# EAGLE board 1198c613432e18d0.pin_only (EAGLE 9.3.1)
REV: F

Size 85.72 x 54.1 mm. Coordinates in mm from the lower left corner, seen from the top.
Outline: 0,51.05 0,3.17 arc90 3.05,0 82.68,0 arc90 85.72,3.17 85.72,51.05 arc90 82.68,54.1 60.77,54.1 59.37,52.71 56.07,52.71 54.67,54.1 3.05,54.1 arc90 0,51.05
Copper layers (1*16): Top 0.035mm / dielectric 1.5mm / Bottom 0.035mm
Design rules "adafruit *": minimum track width 8mil, minimum drill 19mil, track to track 8mil, track to pad 8mil, pad to pad 8mil, via to via 8mil, smd to smd 8mil, copper to edge 10mil, drill to drill 8mil, minimum pad ring 10mil, minimum via ring 8mil, stop-mask expansion 2mil, vias tented up to drill 20mil, thermal gap 10mil
Net classes: 1 power: width 0.305 mm; 2 gnd: width 0.254 mm

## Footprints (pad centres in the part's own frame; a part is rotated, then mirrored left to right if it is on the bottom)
6MM_SMT = smd 2 x 1.2: A -3.3,-2.2; A' 3.3,-2.2; B -3.3,2.2; B' 3.3,2.2
0603-NO = smd 1.075 x 1: 1 -0.85,0; 2 0.85,0
0805-NO = smd 1.24 x 1.5: 1 -0.95,0; 2 0.95,0
_0805MP = smd 1.2 x 1.3: 1 -1.016,0; 2 1.016,0
CHIPLED_0805_NOOUTLINE = smd 1.2 x 1.2: A 0,-1.05; C 0,1.05
SOD-323 = smd 1.35 x 0.8: A 1.27,0; C -1.27,0
SOD-123 = smd 1.4 x 1.4: A 1.85,0; C -1.85,0
JSTPH4 = smd 1 x 4.6: 1 -3,-3.7; 2 -1,-3.7; 3 1,-3.7; 4 3,-3.7 | smd 1.7 x 3.4: NC1 -5.7,1.5; NC2 5.7,1.5
TSSOP16 = smd 0.305 x 0.991: 1 -2.275,-2.918; 2 -1.625,-2.918; 3 -0.975,-2.918; 4 -0.325,-2.918; 5 0.325,-2.918; 6 0.975,-2.918; 7 1.625,-2.918; 8 2.275,-2.918; 9 2.275,2.918; 10 1.625,2.918; 11 0.975,2.918; 12 0.325,2.918; 13 -0.325,2.918; 14 -0.975,2.918; 15 -1.625,2.918; 16 -2.275,2.918
SOT23-6 = smd 0.55 x 1.2: 1 -0.95,-1.3; 2 0,-1.3; 3 0.95,-1.3; 4 0.95,1.3; 5 0,1.3; 6 -0.95,1.3
LGA16_3X3MM = smd 0.5 x 0.25: 1 -1.35,1; 2 -1.35,0.5; 3 -1.35,0; 4 -1.35,-0.5; 5 -1.35,-1; 9 1.35,-1; 10 1.35,-0.5; 11 1.35,0; 12 1.35,0.5; 13 1.35,1 | smd 0.25 x 0.5: 6 -0.5,-1.35; 7 0,-1.35; 8 0.5,-1.35; 14 0.5,1.35; 15 0,1.35; 16 -0.5,1.35
JD-T1800 = smd 0.5 x 2: 1 5.2,-13.1; 2 4.4,-13.1; 3 3.6,-13.1; 4 2.8,-13.1; 5 2,-13.1; 6 1.2,-13.1; 7 0.4,-13.1; 8 -0.4,-13.1; 9 -1.2,-13.1; 10 -2,-13.1; 11 -2.8,-13.1; 12 -3.6,-13.1; 13 -4.4,-13.1; 14 -5.2,-13.1 | hole 0.6: -12.8,-16.9; 7.65,-16.9
LED3535 = smd 1 x 0.85: 1 -1.75,0.875; 2 -1.75,-0.875; 3 1.75,-0.875; 4 1.75,0.875
FEATHERWING_SMT_NOHOLES = smd 1.524 x 2.54: 1 6.35,2.413; 1B 6.35,-2.413; 2 8.89,2.413; 2B 8.89,-2.413; 15 41.91,2.413; 15B 41.91,-2.413; 16 44.45,2.413; 16B 44.45,-2.413; 17 44.45,20.447; 17B 44.45,25.273; 18 41.91,20.447; 18B 41.91,25.273; 27 19.05,20.447; 27B 19.05,25.273; 28 16.51,20.447; 28B 16.51,25.273 | smd 1.524 x 3.048: 3 11.43,2.159; 3B 11.43,-2.159; 4 13.97,2.159; 4B 13.97,-2.159; 5 16.51,2.159; 5B 16.51,-2.159; 6 19.05,2.159; 6B 19.05,-2.159; 7 21.59,2.159; 7B 21.59,-2.159; 8 24.13,2.159; 8B 24.13,-2.159; 9 26.67,2.159; 9B 26.67,-2.159; 10 29.21,2.159; 10B 29.21,-2.159; 11 31.75,2.159; 11B 31.75,-2.159; 12 34.29,2.159; 12B 34.29,-2.159; 13 36.83,2.159; 13B 36.83,-2.159; 14 39.37,2.159; 14B 39.37,-2.159; 19 39.37,20.701; 19B 39.37,25.019; 20 36.83,20.701; 20B 36.83,25.019; 21 34.29,20.701; 21B 34.29,25.019; 22 31.75,20.701; 22B 31.75,25.019; 23 29.21,20.701; 23B 29.21,25.019; 24 26.67,20.701; 24B 26.67,25.019; 25 24.13,20.701; 25B 24.13,25.019; 26 21.59,20.701; 26B 21.59,25.019
JSTPH3 = smd 1 x 4.6: 1 -2,-2.7; 2 0,-2.7; 3 2,-2.7 | smd 1.6 x 3.4: NC1 -4.4,2.5; NC2 4.4,2.5
SOT23-R = smd 0.635 x 1.016: 1 -0.95,-1; 2 0.95,-1; 3 0,1
SOT23-WIDE = smd 1 x 1.2: 1 -0.95,-1; 2 0.95,-1; 3 0,1
SOT363 = smd 0.5 x 0.5: 1 -0.75,-0.9; 3 0.75,-0.9; 4 0.75,0.9; 6 -0.75,0.9 | smd 0.4 x 0.5: 2 0,-0.9; 5 0,0.9
RESPACK_4X0603 = smd 0.45 x 0.9: 1 -1.3,-0.85; 2 -0.4,-0.85; 3 0.4,-0.85; 4 1.3,-0.85; 5 1.3,0.85; 6 0.4,0.85; 7 -0.4,0.85; 8 -1.3,0.85
SOLDERJUMPER_2WAY_OPEN_NOPASTE = smd 1.168 x 1.6: 1 -1.397,0; 2 0,0; 3 1.397,0
SOLDERJUMPER_CLOSEDWIRE = smd 1.168 x 1.6: 1 -0.762,0; 2 0.762,0 | smd 0.635 x 0.203: WIRE 0,0
BUZZER_SMT_7.5MM = smd 2 x 2: + 2.8,-2.8; - 2.8,2.8; MT2 -2.8,2.8 | smd 2 x 1 rotated 135: MT -3,-3
EVQ-Q2_SMALLER = smd 2 x 1.2: A -3.1,-2; A' 3.1,-2; B -3.1,2; B' 3.1,2
SPDT_SMT_SSSS811101 = smd 0.7 x 1.5: A -2.25,1.75; B 0.75,1.75; C 2.25,1.75 | smd 1 x 0.8: SUP1 -3.65,1.1; SUP2 -3.65,-1.1; SUP3 3.65,1.1; SUP4 3.65,-1.1 | hole 0.9: -1.5,0; 1.5,0
TESTPOINT_ROUND_2MM = smd 2 x 2: P$1 0,0
SOIC8_208MIL = smd 0.6 x 2.2: 1 -1.905,-3.315; 2 -0.635,-3.315; 3 0.635,-3.315; 4 1.905,-3.315; 5 1.905,3.315; 6 0.635,3.315; 7 -0.635,3.315; 8 -1.905,3.315
SOT23-5 = smd 0.55 x 1.2: 1 -0.95,-1.3; 2 0,-1.3; 3 0.95,-1.3; 4 0.95,1.3; 5 -0.95,1.3
ALS-PT26-21C = smd 1.5 x 1.6: 1_E -1.8,0; 2_C 1.8,0 | hole 2.4: 0,0
MOUNTINGHOLE_3.0_PLATEDTHIN = drill 3 pad 3.6: P$1 0,0
53398-0271 = smd 0.8 x 1.6: 1 0.625,-1.27; 2 -0.625,-1.27 | smd 2.1 x 3: M1 3.185,1.48; M2 -3.185,1.48
PQFN64-1 = smd 0.7 x 0.22: 1 -4.45,3.75; 2 -4.45,3.25; 3 -4.45,2.75; 4 -4.45,2.25; 5 -4.45,1.75; 6 -4.45,1.25; 7 -4.45,0.75; 8 -4.45,0.25; 9 -4.45,-0.25; 10 -4.45,-0.75; 11 -4.45,-1.25; 12 -4.45,-1.75; 13 -4.45,-2.25; 14 -4.45,-2.75; 15 -4.45,-3.25; 16 -4.45,-3.75; 33 4.45,-3.75; 34 4.45,-3.25; 35 4.45,-2.75; 36 4.45,-2.25; 37 4.45,-1.75; 38 4.45,-1.25; 39 4.45,-0.75; 40 4.45,-0.25; 41 4.45,0.25; 42 4.45,0.75; 43 4.45,1.25; 44 4.45,1.75; 45 4.45,2.25; 46 4.45,2.75; 47 4.45,3.25; 48 4.45,3.75 | smd 0.22 x 0.7: 17 -3.75,-4.45; 18 -3.25,-4.45; 19 -2.75,-4.45; 20 -2.25,-4.45; 21 -1.75,-4.45; 22 -1.25,-4.45; 23 -0.75,-4.45; 24 -0.25,-4.45; 25 0.25,-4.45; 26 0.75,-4.45; 27 1.25,-4.45; 28 1.75,-4.45; 29 2.25,-4.45; 30 2.75,-4.45; 31 3.25,-4.45; 32 3.75,-4.45; 49 3.75,4.45; 50 3.25,4.45; 51 2.75,4.45; 52 2.25,4.45; 53 1.75,4.45; 54 1.25,4.45; 55 0.75,4.45; 56 0.25,4.45; 57 -0.25,4.45; 58 -0.75,4.45; 59 -1.25,4.45; 60 -1.75,4.45; 61 -2.25,4.45; 62 -2.75,4.45; 63 -3.25,4.45; 64 -3.75,4.45 | smd 4.7 x 4.7: EXP 0,0
FIDUCIAL_1MM = smd 1 x 1: 1 0,0
JSTPH2 = smd 1 x 4.6: 1 -1,-3.7; 2 1,-3.7 | smd 1.6 x 3.4: NC1 -3.4,1.5; NC2 3.4,1.5
2X05_1.27MM_BOX_POSTS = smd 0.76 x 2.6: 1 -2.54,-2.15; 2 -2.54,2.15; 3 -1.27,-2.15; 4 -1.27,2.15; 5 0,-2.15; 6 0,2.15; 7 1.27,-2.15; 8 1.27,2.15; 9 2.54,-2.15; 10 2.54,2.15 | hole 1: -1.905,0; 1.905,0
4UCONN_20329_V2 = smd 1 x 2: BASE@1 -0.75,-2; BASE@2 0.75,-2 | smd 0.4 x 1.35: D+ 0,0.775; D- -0.65,0.775; GND 1.3,0.775; ID 0.65,0.775; VBUS -1.3,0.775 | drill 0.8 pad 1.143 offset: SPRT@1 -3.3,0.9; SPRT@2 3.3,0.9 | drill 0.9 pad 2.413 square: SPRT@3 -3.6,-1.9; SPRT@4 3.6,-1.9 | hole 0.7: -1.95,0; 1.95,0

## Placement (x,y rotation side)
A  [6MM_SMT]  5.14,34.93 270 bottom
B  [6MM_SMT]  12.83,30.04 270 bottom
C1  1uF  [0603-NO]  77.47,52.77 0 top
C2  1uF  [0603-NO]  48.64,9.08 0 top
C3  10µF  [0805-NO]  42.29,37.21 180 top
C4  1uF  [0603-NO]  26.35,16.26 90 top
C5  10uF  [0805-NO]  36.51,45.21 270 top
C6  10µF  [0805-NO]  41.72,44.39 180 top
C7  1uF  [0603-NO]  44.66,38.34 90 top
C8  10µF  [0805-NO]  45.23,35.12 270 top
C9  0.1uF  [0603-NO]  17.97,45.34 180 top
C10  10uF  [0805-NO]  68.01,2.16 0 top
C11  10uF  [0805-NO]  26.23,30.72 270 top
C12  1uF  [0603-NO]  37.08,19.49 180 top
C13  1uF  [0603-NO]  26.42,41.66 270 top
C14  10uF  [0805-NO]  48.7,17.34 270 top
C15  10uF  [0805-NO]  16.51,52.64 0 top
C16  10µF  [_0805MP]  25.55,36.78 180 top
C17  0.1uF  [0603-NO]  23.81,12.89 0 top
C18  10uF  [0805-NO]  42.1,35.37 180 top
C19  1uF  [0603-NO]  42.16,33.85 180 top
CHG  ORANGE  [CHIPLED_0805_NOOUTLINE]  36.58,52.07 180 top
D1  3.6V  [SOD-323]  24.51,10.54 0 top
D2  3.6V  [SOD-323]  68.26,5.78 270 top
D4  MBR0540  [SOD-123]  46.48,47.12 0 top
DOWN  [6MM_SMT]  74.93,27.18 45 bottom
FB1  Ferrite  [0805-NO]  26.48,44.96 270 top
I2C  JST PH 4  [JSTPH4]  42.86,3.49 180 top
IC1  74165TSSOP  [TSSOP16]  71.69,50.23 270 top
IC2  PAM8301  [SOT23-6]  16.19,49.72 0 top
IC4  LIS3DH  [LGA16_3X3MM]  47.75,11.75 180 top
L  RED  [CHIPLED_0805_NOOUTLINE]  48.98,51.97 0 top
LCD1  DISP_LCD_JDT1800  [JD-T1800]  40.13,28.83 90 bottom
LED1  WS2812B3535  [LED3535]  60.33,6.48 0 bottom
LED2  WS2812B3535  [LED3535]  51.59,6.48 0 bottom
LED3  WS2812B3535  [LED3535]  42.86,6.48 0 bottom
LED4  WS2812B3535  [LED3535]  34.13,6.48 0 bottom
LED5  WS2812B3535  [LED3535]  25.4,6.48 0 bottom
LEFT  [6MM_SMT]  80.2,32.51 315 bottom
MS1  FEATHERWING_SMTDUALNOHOLES  [FEATHERWING_SMT_NOHOLES]  31.43,54.1 270 top
NEOPIX  JST PH 3  [JSTPH3]  24.64,4.51 180 top
Q1  DMG3405  [SOT23-R]  45.85,41.66 180 top
Q2  DMG3405  [SOT23-R]  45.85,44.45 180 top
Q3  BSS138  [SOT23-WIDE]  24.08,34.24 90 top
Q4  BSS138  [SOT363]  53.53,3.56 0 top
R1  100K  [RESPACK_4X0603]  47.62,34.04 90 top
R2  1K  [0603-NO]  36.58,48.77 270 top
R3  10K  [0603-NO]  28,49.85 0 top
R4  10K  [RESPACK_4X0603]  53.59,6.54 0 top
R5  1K  [0603-NO]  21.15,9.72 90 top
R6  1K  [0603-NO]  66.93,6.6 90 top
R7  2.2K  [0603-NO]  50.04,49.02 180 top
R8  4.7K  [0603-NO]  41.59,42.86 0 top
R9  DNP  [0603-NO]  52.58,9.14 0 bottom
R10  100K  [RESPACK_4X0603]  77.47,50.04 270 top
R11  100K  [RESPACK_4X0603]  66.48,50.29 90 top
R12  47K  [0603-NO]  17.59,46.86 0 top
R14  10K  [0603-NO]  24.7,15.24 270 top
R15  10K  [0603-NO]  26.29,12.83 270 top
R16  10  [0603-NO]  23.62,30.99 90 top
R17  100K  [0603-NO]  26.45,34.12 90 top
R19  100K  [0603-NO]  37.08,17.97 180 top
RIGHT  [6MM_SMT]  69.66,32.51 135 bottom
SELECT  [6MM_SMT]  73.22,50.42 180 bottom
SENSE  JST PH 3  [JSTPH3]  61.02,4.51 180 top
SJ1  [SOLDERJUMPER_2WAY_OPEN_NOPASTE]  70.87,4.25 270 top
SJ2  [SOLDERJUMPER_CLOSEDWIRE]  13.84,44.58 180 top
SP1  SPEAKER_7.5MM  [BUZZER_SMT_7.5MM]  10.16,49.59 270 top
START  [6MM_SMT]  12.76,50.42 180 bottom
SW1  SPST_TACT-EVQQ2  [EVQ-Q2_SMALLER]  22.48,50.48 0 top
SW11  [SPDT_SMT_SSSS811101]  57.78,51.24 180 top
TP6  [TESTPOINT_ROUND_2MM]  9.91,10.73 0 top
TP7  [TESTPOINT_ROUND_2MM]  5.14,10.79 0 top
TP8  [TESTPOINT_ROUND_2MM]  13.65,10.86 0 top
U1  GD25Q16  [SOIC8_208MIL]  40.26,13.72 270 top
U2  AP2112-3.3  [SOT23-5]  47.37,38.23 90 top
U3  MCP73831T-2ACI/OT  [SOT23-5]  42.29,40.13 0 top
U4  ALS-PT21  [ALS-PT26-21C]  30.03,51.8 0 top
U$5  MOUNTINGHOLE3.0THIN  [MOUNTINGHOLE_3.0_PLATEDTHIN]  3.81,50.29 0 top
U$6  MOUNTINGHOLE3.0THIN  [MOUNTINGHOLE_3.0_PLATEDTHIN]  81.92,50.29 0 top
U$8  [SPEAKER_OVAL8OHM]  12.13,25.27 90 top
U$13  CON_MOLEX_2P  [53398-0271]  22.67,41.59 90 top
U$15  MOUNTINGHOLE3.0THIN  [MOUNTINGHOLE_3.0_PLATEDTHIN]  3.81,3.94 0 top
U$17  MOUNTINGHOLE3.0THIN  [MOUNTINGHOLE_3.0_PLATEDTHIN]  81.92,3.94 0 top
U$18  [PYBADGE_TOP]  85.72,0.13 0 bottom
U$24  ATSAMD51J19  [PQFN64-1]  42.61,25.4 0 top
U$32  [PYBADGE_BOT]  0,0.13 0 top
U$34  FIDUCIAL_1MM  [FIDUCIAL_1MM]  1.52,7.24 270 top
U$35  FIDUCIAL_1MM  [FIDUCIAL_1MM]  84.18,47.51 270 top
U$37  [PCBFEAT-REV-040]  37.21,9.4 0 top
U$42  FIDUCIAL_1MM  [FIDUCIAL_1MM]  83.95,46.67 0 bottom
U$43  FIDUCIAL_1MM  [FIDUCIAL_1MM]  7.24,1.4 0 bottom
UP  [6MM_SMT]  74.93,37.85 225 bottom
X1  JSTPH  [JSTPH2]  54.1,43.31 270 top
X2  2x5 0.05" SWD  [2X05_1.27MM_BOX_POSTS]  9.33,5.14 0 top
X3  microUSB  [4UCONN_20329_V2]  42.86,49.91 180 top

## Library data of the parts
A B C1-C7 C9-C19 CHG D1 D2 D4 DOWN FB1 I2C IC1 IC2 IC4 L LCD1 LED1-LED5 LEFT MS1 NEOPIX Q1-Q4 R1-R12 R14-R17 R19 RIGHT SELECT SENSE SJ1 SJ2 SP1 START SW1 SW11 TP6-TP8 U1-U4 U$8 U$13 U$24 U$37 UP X1-X3 = microbuilder
C8 = microbuilder; COMPANY: ADAFRUIT INDUSTRIES; DRAWN: KTOWN; REV: A
U$5 U$6 U$15 U$17 U$34 U$35 U$42 U$43 = microbuilder; BOM: EXCLUDE
U$18 U$32 = feather_silks

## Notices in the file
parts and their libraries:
microbuilder: This work is placed in the public domain, and may be freely used for commercial and non-commercial work with the following conditions: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
